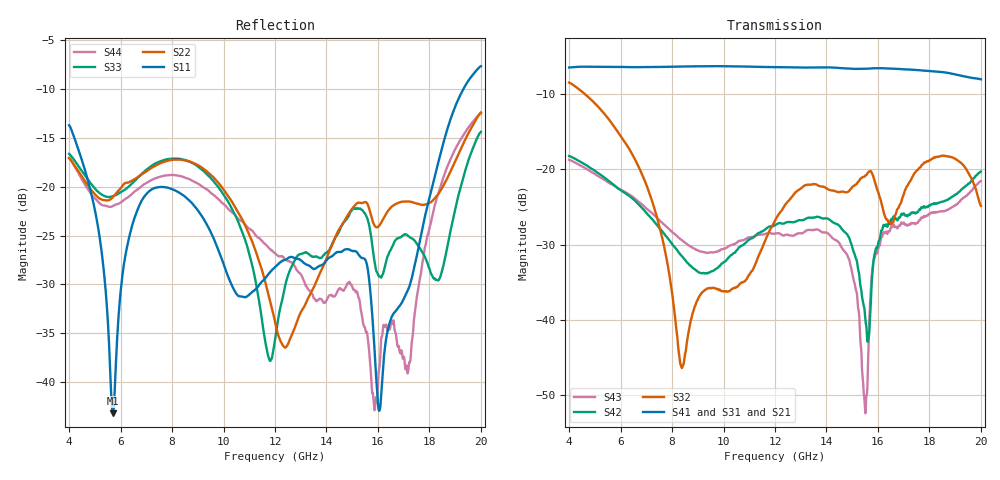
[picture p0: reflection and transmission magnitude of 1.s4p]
!Keysight Technologies,N5247B,US57180241,A.12.85.04
!Date: Friday, March 23, 2018 09:45:48
!Correction: S11(Full 4 Port(1,2,3,4))
!S12(Full 4 Port(1,2,3,4))
!S13(Full 4 Port(1,2,3,4))
!S14(Full 4 Port(1,2,3,4))
!S21(Full 4 Port(1,2,3,4))
!S22(Full 4 Port(1,2,3,4))
!S23(Full 4 Port(1,2,3,4))
!S24(Full 4 Port(1,2,3,4))
!S31(Full 4 Port(1,2,3,4))
!S32(Full 4 Port(1,2,3,4))
!S33(Full 4 Port(1,2,3,4))
!S34(Full 4 Port(1,2,3,4))
!S41(Full 4 Port(1,2,3,4))
!S42(Full 4 Port(1,2,3,4))
!S43(Full 4 Port(1,2,3,4))
!S44(Full 4 Port(1,2,3,4))
!S4P File: Measurements: <S11,S12,S13,S14>,
!<S21,S22,S23,S24>,
!<S31,S32,S33,S34>,
!<S41,S42,S43,S44>:
# Hz S  dB  R 50
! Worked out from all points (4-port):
!   6401 points, 4 GHz to 20 GHz, reference 50 ohm
!   strongest paths, dB at 4 GHz, 8 GHz, 12 GHz, 16 GHz, 20 GHz:
!     S41: -6.4, -6.3, -6.4, -6.5, -8.0
!     S31: -6.5, -6.3, -6.5, -6.7, -7.9
!     S21: -6.4, -6.5, -6.6, -6.2, -8.4
!     S32: -8.4, -36.4, -26.8, -22.9, -24.8
!     S42: -18.2, -29.9, -27.4, -30.0, -20.3
!     S43: -18.7, -28.3, -28.6, -30.7, -21.5
!   lowest |S11| = -43.2 dB at 5.697 GHz (marker M1), VSWR 1.01, Z = 50.5 + j0.428 ohm
!   |S11| at or under -10 dB: start of sweep to 19.32 GHz
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4e9  -13.70 22.4  -6.45 -147.6  -6.54 -149.3  -6.41 -148.6
     -6.41 -147.4  -17.08 -24.0  -8.44 -121.4  -18.16 119.8
     -6.49 -149.3  -8.43 -121.6  -16.63 -25.7  -18.66 118.2
     -6.41 -148.7  -18.22 119.5  -18.72 118.1  -17.03 -23.5
5.6975e9  -43.19 37.7  -6.22 142.8  -6.26 140.9  -6.31 141.9
          -6.21 142.9  -21.07 -31.8  -14.04 -176.4  -21.90 22.9
          -6.26 141.0  -14.05 -176.5  -20.97 -38.7  -22.03 17.7
          -6.34 141.8  -21.94 22.7  -22.06 17.6  -21.97 -31.4
8.3825e9  -20.77 -17.9  -6.52 31.6  -6.39 30.0  -6.27 31.5
          -6.46 31.7  -17.24 -88.7  -46.46 -172.2  -31.46 -163.1
          -6.32 29.8  -46.46 -172.1  -17.18 -88.7  -29.33 -169.0
          -6.29 31.5  -31.55 -163.2  -29.41 -168.8  -18.94 -94.3
1.444e10  -26.67 0.7  -6.57 121.4  -6.70 118.6  -6.42 119.5
          -6.58 121.5  -24.60 -16.1  -23.06 -126.5  -27.31 86.1
          -6.67 117.6  -23.02 -127.5  -24.82 -38.8  -29.51 86.7
          -6.46 119.1  -27.34 85.6  -29.57 87.3  -30.64 7.2
1.55125e10  -27.49 -54.1  -6.09 68.8  -6.65 65.1  -6.52 66.0
            -6.15 69.5  -21.56 -57.6  -20.85 -140.9  -39.98 32.2
            -6.66 65.7  -20.81 -141.0  -22.81 -77.7  -52.88 -50.0
            -6.58 67.2  -39.99 32.7  -52.49 -49.5  -34.68 -66.5
1.60525e10  -42.92 -37.2  -6.31 36.8  -6.95 37.2  -6.63 39.0
            -6.26 36.8  -23.97 -60.6  -23.73 -171.5  -29.51 67.6
            -6.69 37.8  -23.52 -171.0  -29.18 -70.7  -30.07 82.4
            -6.51 39.5  -29.45 68.0  -30.23 82.4  -38.63 79.9
2e10  -7.65 59.0  -8.11 -179.7  -7.95 -176.5  -8.03 -174.3
      -8.39 179.9  -12.39 66.4  -25.16 146.2  -20.59 157.5
      -7.88 -178.8  -24.84 144.3  -14.38 47.9  -21.50 154.9
      -7.99 -176.1  -20.26 156.2  -21.54 155.4  -12.48 54.1
